{attribute 'pack_mode' := '1'}
TYPE ST_B_To_A :
STRUCT
    SequenceNo  : UDINT;
    Running     : BOOL;
    ActualValue : REAL;
    AlarmCode   : INT;
	Hello : STRING := 'Hello from B to A';
END_STRUCT
END_TYPE
